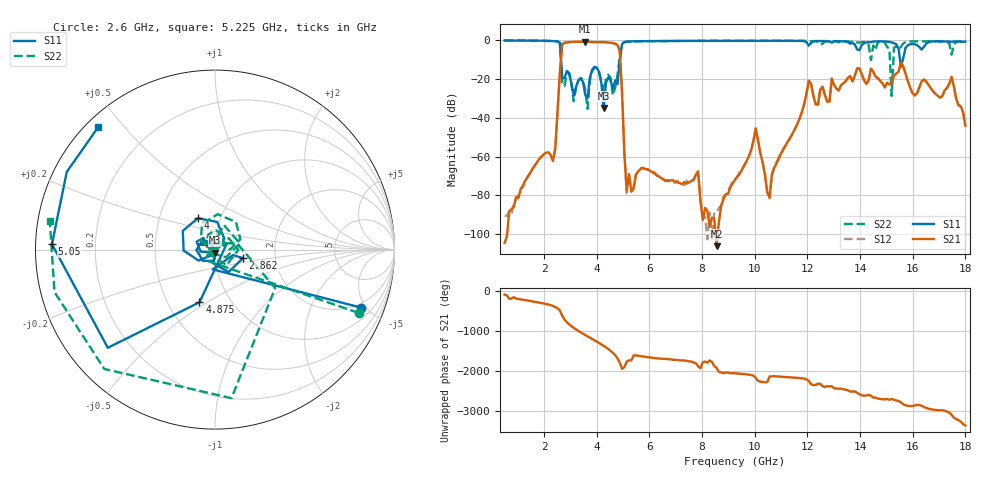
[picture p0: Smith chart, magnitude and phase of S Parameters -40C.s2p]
!Agilent Technologies,N5230A,MY45001468,A.07.50.67
!Agilent N5230A: A.07.50.67
!Date: Thursday, June 27, 2024 16:38:21
!Correction: S11(Full 2 Port(1,2))
!S21(Full 2 Port(1,2))
!S12(Full 2 Port(1,2))
!S22(Full 2 Port(1,2))
!S2P File: Measurements: S11, S21, S12, S22:
# Hz S  dB  R 50
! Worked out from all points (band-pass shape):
!   201 points, 500 MHz to 18 GHz, reference 50 ohm
!   highest |S21| = -0.66 dB at 3.562 GHz (marker M1); lowest = -106.2 dB at 8.55 GHz (marker M2)
!   |S21| within 3 dB of the highest: 2.678 GHz to 4.822 GHz (2.144 GHz wide, 57.2 % of centre)
!   lowest |S11| = -34.9 dB at 4.263 GHz (marker M3), VSWR 1.04, Z = 49.8 - j1.79 ohm
!   |S11| at or under -10 dB: 2.643 GHz to 4.878 GHz (2.235 GHz wide, 59.4 % of centre); 15.52 GHz to 15.62 GHz (107.4 MHz wide, 0.69 % of centre)
!   |S22| runs from -35.3 to 0.0 dB; largest |S21 - S12| = 0.0042
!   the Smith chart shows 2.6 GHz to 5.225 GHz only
!   S11 on the Smith chart (normalised r, x): 2.6 GHz: 1.69, -4.64; 2.862 GHz: 1.36, -0.13; 4 GHz: 0.78, +0.28; 4.875 GHz: 0.72, -0.46; 5.05 GHz: 0.05, +0.02; 5.225 GHz: 0.03, +0.43
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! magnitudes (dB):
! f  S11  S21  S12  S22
! 500 MHz  0.0  -104.5  -90.4  0.0
! 2.337 GHz  -0.3  -62.3  -62.0  -0.3
! 2.6 GHz  -1.2  -16.5  -16.5  -1.2
! 2.862 GHz  -15.7  -1.0  -1.1  -16.7
! 3.475 GHz  -21.2  -0.7  -0.7  -20.4
! 3.562 GHz  -28.0  -0.7  -0.7  -25.7
! 4 GHz  -14.0  -0.9  -0.9  -14.3
! 4.263 GHz  -34.9  -0.9  -0.9  -26.5
! 4.875 GHz  -10.3  -5.5  -5.6  -8.0
! 5.05 GHz  -0.8  -58.6  -58.7  -0.8
! 5.225 GHz  -0.5  -69.0  -69.3  -0.6
! 6.362 GHz  -0.3  -70.2  -70.6  -0.3
! 8.55 GHz  -0.2  -106.2  -88.7  -0.2
! 9.25 GHz  -0.2  -72.0  -71.7  -0.2
! 10.04 GHz  -0.2  -45.4  -45.5  -0.2
! 10.56 GHz  -0.2  -81.1  -81.6  -0.2
! 12.22 GHz  -0.5  -28.5  -28.6  -0.4
! 15.11 GHz  -0.7  -22.7  -22.8  -4.2
! 15.2 GHz  -1.0  -22.1  -22.3  -28.6
! 15.29 GHz  -1.4  -18.1  -18.2  -3.8
! 17.48 GHz  -0.7  -18.7  -18.9  -7.3
! 18 GHz  -0.6  -43.9  -44.4  -0.4
